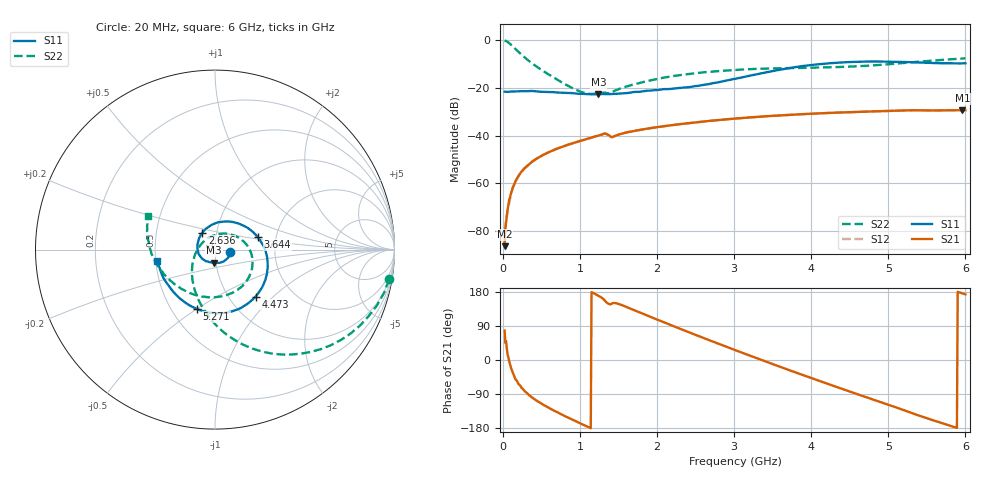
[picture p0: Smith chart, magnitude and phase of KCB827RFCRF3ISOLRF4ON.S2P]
!Agilent Technologies,E5071B,JP1KK00126,A.08.11
!Date: Tue May 06 07:21:08 2014
!Data & Calibration Information:
!Freq	S11:SOLT2(ON)	S21:SOLT2(ON)	S12:SOLT2(ON)	S22:SOLT2(ON)
# Hz S dB R 50
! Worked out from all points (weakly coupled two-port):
!   600 points, 20 MHz to 6 GHz, reference 50 ohm
!   highest |S21| = -29.36 dB at 5.96 GHz (marker M1); lowest = -86.4 dB at 20 MHz (marker M2)
!   lowest |S11| = -22.7 dB at 1.238 GHz (marker M3), VSWR 1.16, Z = 48.9 - j7.17 ohm
!   |S11| at or under -10 dB: start of sweep to 4.128 GHz
!   |S22| runs from -22.6 to -0.1 dB; largest |S21 - S12| = 0.00021
!   S11 on the Smith chart (normalised r, x): 20 MHz: 1.18, -0.04; 2.636 GHz: 0.85, +0.16; 3.644 GHz: 1.60, +0.24; 4.473 GHz: 1.32, -0.78; 5.271 GHz: 0.67, -0.50; 6 GHz: 0.51, -0.07
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2e7  -21.60 -10.5  -86.35 77.7  -84.94 50.5  -0.13 -9.6
3.996661e7  -21.65 -7.1  -76.39 49.4  -74.65 49.9  -0.40 -18.9
7.989983e7  -21.60 -7.8  -66.81 -3.9  -68.36 -4.6  -1.27 -35.6
1.098498e8  -21.55 -9.6  -63.52 -24.8  -63.54 -22.3  -2.12 -46.6
1.797329e8  -21.42 -14.5  -57.88 -55.1  -58.25 -56.3  -4.28 -66.9
2.595993e8  -21.39 -21.0  -54.37 -77.4  -54.40 -77.2  -6.65 -83.8
3.694157e8  -21.30 -31.4  -51.19 -98.2  -51.15 -97.5  -9.56 -101.6
5.09182e8  -21.64 -43.1  -48.34 -116.4  -48.32 -116.6  -12.72 -121.2
1.018331e9  -22.47 -80.4  -42.09 -168.8  -42.05 -168.7  -21.77 157.0
1.237963e9  -22.73 -94.4  -39.97 169.2  -40.00 169.2  -22.44 107.9
1.327813e9  -22.61 -99.9  -39.19 154.9  -39.19 155.0  -22.03 88.4
1.427646e9  -22.54 -106.9  -40.47 150.3  -40.50 150.0  -21.50 79.1
2.016661e9  -20.85 -157.5  -36.39 105.3  -36.42 105.2  -16.19 21.7
2.635626e9  -18.60 127.3  -33.99 55.3  -34.01 55.3  -13.41 -13.5
3.014992e9  -16.18 80.6  -32.86 26.0  -32.89 25.8  -12.48 -33.2
3.64394e9  -12.10 16.3  -31.44 -21.5  -31.45 -21.6  -11.75 -65.8
4.013322e9  -10.37 -14.3  -30.83 -48.5  -30.83 -48.6  -11.57 -87.7
4.472554e9  -9.23 -49.2  -30.22 -81.4  -30.22 -81.5  -11.14 -117.3
5.011653e9  -9.00 -87.9  -29.67 -118.9  -29.66 -119.1  -10.05 -153.3
5.271219e9  -9.23 -107.0  -29.41 -137.4  -29.40 -137.6  -9.36 -169.0
5.960067e9  -9.75 -164.9  -29.36 176.0  -29.35 175.8  -7.70 155.3
6e9  -9.69 -168.8  -29.38 173.2  -29.36 173.1  -7.63 153.6
